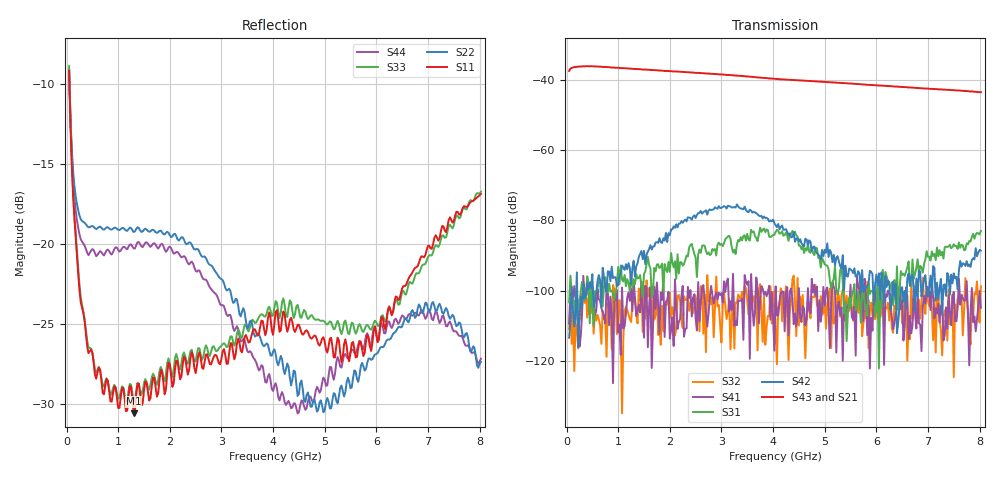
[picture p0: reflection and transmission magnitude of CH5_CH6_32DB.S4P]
!Agilent Technologies,E5071C,MY46316741,A.11.02
!Date: Mon Jun 01 10:41:50 2026
!Data & Calibration Information:
!1:CH5 INPUT 2:CH5 OUTPUT 3:CH6 INPUT 4:CH6 OUTPUT
!Freq	S11:SOLT4(ON)	S12:SOLT4(ON)	S13:SOLT4(ON)	S14:SOLT4(ON)
!	S21:SOLT4(ON)	S22:SOLT4(ON)	S23:SOLT4(ON)	S24:SOLT4(ON)
!	S31:SOLT4(ON)	S32:SOLT4(ON)	S33:SOLT4(ON)	S34:SOLT4(ON)
!	S41:SOLT4(ON)	S42:SOLT4(ON)	S43:SOLT4(ON)	S44:SOLT4(ON)
!PortZ  Port1:50+j0  Port2:50+j0  Port3:50+j0  Port4:50+j0
!Above PortZ is port z conversion or system Z0 setting when saving the data.
!When reading, reference impedance value at option line is always used.
# Hz S dB R 50
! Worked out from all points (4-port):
!   320 points, 50 MHz to 8.025 GHz, reference 50 ohm
!   strongest paths, dB at 50 MHz, 2.05 GHz, 4.05 GHz, 6.05 GHz, 8.025 GHz:
!     S43: -37.4, -37.5, -39.7, -41.6, -43.5
!     S21: -37.4, -37.6, -39.8, -41.8, -43.7
!     S42: -113.4, -82.6, -81.4, -95.1, -88.7
!     S31: -103.3, -92.1, -83.3, -122.2, -83.0
!     S41: -109.3, -107.6, -98.8, -100.9, -104.9
!     S32: -111.0, -104.7, -110.0, -102.4, -98.8
!   lowest |S11| = -30.6 dB at 1.3 GHz (marker M1), VSWR 1.06, Z = 47.7 - j1.81 ohm
!   |S11| at or under -10 dB: 56.21 MHz to end of sweep
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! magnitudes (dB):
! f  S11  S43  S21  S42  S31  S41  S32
! 50 MHz  -9.2  -37.4  -37.4  -113.4  -103.3  -109.3  -111.0
! 175 MHz  -19.5  -36.3  -36.3  -106.0  -109.0  -101.5  -109.5
! 400 MHz  -26.4  -36.1  -36.1  -97.8  -95.9  -98.5  -107.7
! 1.3 GHz  -30.6  -36.9  -36.9  -91.5  -97.1  -96.8  -101.9
! 4.475 GHz  -25.1  -40.1  -40.2  -85.1  -84.6  -106.9  -96.4
! 5.9 GHz  -26.7  -41.4  -41.6  -94.6  -100.1  -107.8  -103.4
! 8.025 GHz  -16.9  -43.5  -43.7  -88.7  -83.0  -104.9  -98.8
